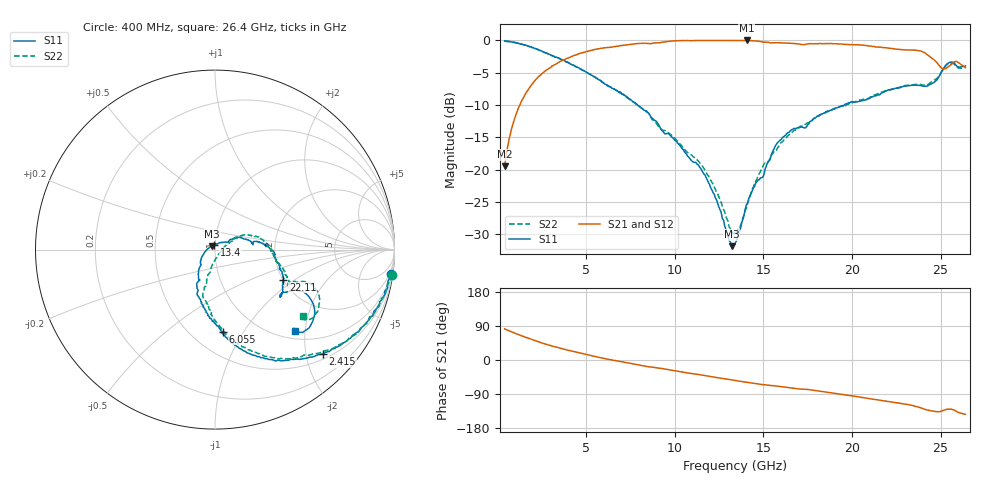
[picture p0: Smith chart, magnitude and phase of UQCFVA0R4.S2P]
!  Part Number  UQCFVA0R4  Mounting Orientation: Horizontal
!  Description: Ultra Low ESR Microwave capacitors
!  Application: Coupling, Bypass, Tuning, DC Block
!  Filters, Matching
# GHZ S DB R 50
! Freq  |S11|  S11 Ph  |S21|  S21 Ph  |S12|  S12 Ph  |S22|  S22 Ph
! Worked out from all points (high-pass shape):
!   401 points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, 400 MHz to 26.4 GHz, reference 50 ohm
!   highest |S21| = 0.00 dB at 14.05 GHz (marker M1); lowest = -19.5 dB at 400 MHz (marker M2)
!   |S21| within 3 dB of the highest: 3.734 GHz to 24.64 GHz (20.9 GHz wide, 147 % of centre)
!   lowest |S11| = -31.8 dB at 13.21 GHz (marker M3), VSWR 1.05, Z = 48.4 + j1.95 ohm
!   |S11| at or under -10 dB: 7.91 GHz to 19.56 GHz (11.65 GHz wide, 84.8 % of centre)
!   |S22| runs from -29.9 to -0.1 dB; largest |S21 - S12| = 0.01
!   S11 on the Smith chart (normalised r, x): 400 MHz: 1, -15; 2.415 GHz: 0.61, -2.34; 6.055 GHz: 0.70, -0.81; 13.4 GHz: 0.99, +0.05; 22.11 GHz: 2.01, -0.81; 26.4 GHz: 1.15, -1.76
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0.4  -0.08 -7.8  -19.48 82.0  -19.47 81.8  -0.05 -8.2
1.18  -0.41 -22.8  -10.44 67.1  -10.47 67.3  -0.45 -22.2
2.415  -1.56 -44.0  -5.36 46.3  -5.35 46.5  -1.57 -42.3
3.585  -2.95 -60.0  -3.17 30.4  -3.21 30.3  -2.92 -58.3
4.755  -4.55 -73.3  -1.92 17.4  -1.94 17.3  -4.53 -70.7
6.055  -6.76 -84.6  -1.15 3.6  -1.09 3.5  -6.64 -83.9
9.11  -13.12 -117.5  -0.37 -21.4  -0.37 -21.4  -13.41 -105.3
11.58  -20.37 -144.0  -0.01 -40.2  -0.01 -40.2  -19.53 -101.9
13.205  -31.83 128.3  -0.01 -52.3  -0.01 -52.1  -29.37 -55.1
13.4  -31.45 98.8  -0.01 -53.9  -0.01 -53.9  -29.55 -34.6
14.05  -25.37 49.9  0.00 -58.7  -0.01 -58.7  -25.99 14.2
14.895  -21.24 28.6  -0.19 -64.7  -0.21 -64.6  -19.88 26.8
15.805  -15.81 23.7  -0.36 -69.2  -0.36 -69.0  -16.60 28.2
17.755  -12.37 10.2  -0.51 -79.7  -0.52 -79.5  -12.39 17.5
20.355  -9.45 -7.6  -0.65 -97.0  -0.63 -96.9  -9.31 -8.8
22.11  -7.63 -23.7  -1.22 -109.9  -1.20 -109.7  -7.66 -19.3
23.475  -6.90 -34.9  -1.49 -120.8  -1.43 -120.6  -6.85 -25.0
24.125  -7.11 -34.6  -1.94 -130.2  -1.89 -130.2  -6.96 -25.1
24.905  -5.62 -26.0  -3.83 -136.4  -3.80 -136.4  -5.51 -19.7
25.295  -3.82 -30.7  -4.36 -130.9  -4.31 -130.8  -3.92 -24.3
25.75  -3.46 -43.4  -3.33 -131.9  -3.31 -132.1  -3.64 -36.2
26.4  -3.93 -45.8  -4.17 -143.3  -4.16 -143.0  -4.24 -37.4
